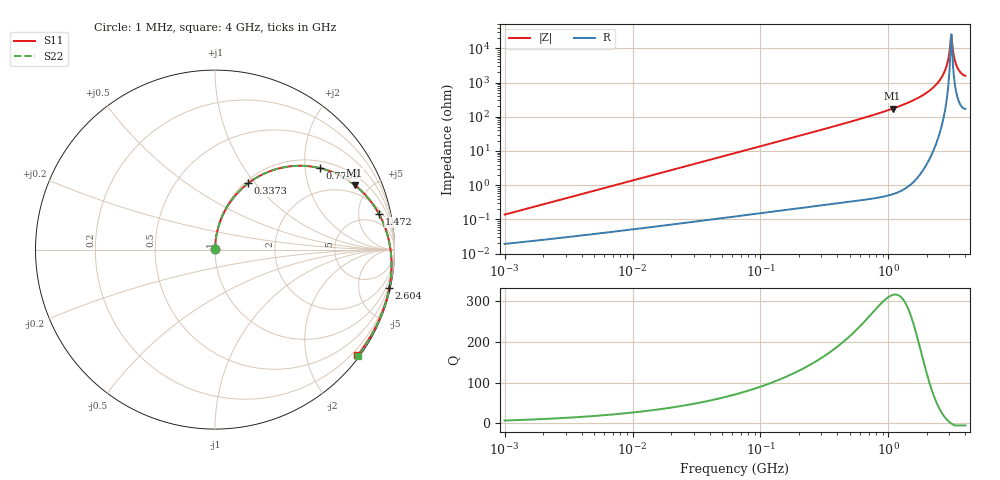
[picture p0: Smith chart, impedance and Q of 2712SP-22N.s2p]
# MHz  S  MA  R  50
!Freq  MagS11  AngS11  MagS21  AngS21  MagS12  AngS12  MagS22  AngS22
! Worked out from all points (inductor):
!   801 points, 1 MHz to 4 GHz, reference 50 ohm
!   read as one part in series: L = 21.9 nH near 1.042 MHz
!   highest Q = 316 at 1.078 GHz (marker M1), where L = 25.4 nH
!   self-resonance near 3.075 GHz
!   S11 on the Smith chart (normalised r, x): 1 MHz: 1.00, +0.00; 337.3 MHz: 1.04, +0.92; 773.6 MHz: 1.20, +2.41; 1.472 GHz: 2.68, +8.46; 2.604 GHz: 0.24, -9.18; 4 GHz: 0.06, -3.02
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1  0.00134 81.6  0.9998 -0.1  0.9998 -0.1  0.00134 81.6
4.016383  0.005336 86.0  0.9996 -0.3  0.9996 -0.3  0.005336 86.0
15.96482  0.02117 87.0  0.9991 -1.3  0.9991 -1.3  0.02116 87.0
63.45894  0.08382 84.0  0.9953 -5.1  0.9953 -5.1  0.08381 84.0
252.2445  0.3189 69.6  0.9455 -20.0  0.9455 -20.0  0.3188 69.6
337.2844  0.4124 63.5  0.9085 -26.2  0.9085 -26.2  0.4123 63.5
543.6043  0.5982 50.1  0.7987 -39.7  0.7987 -39.7  0.598 50.1
773.5614  0.7415 37.7  0.6683 -52.1  0.6683 -52.1  0.7412 37.7
1013.11  0.8378 27.3  0.5436 -62.5  0.5436 -62.5  0.8373 27.3
1078.187  0.8571 24.9  0.5126 -64.9  0.5126 -64.9  0.8567 24.9
1471.91  0.9349 12.3  0.3519 -77.5  0.3519 -77.5  0.9344 12.3
2094.561  0.9834 -2.6  0.1716 -92.0  0.1716 -92.0  0.9832 -2.6
2604.497  0.9945 -12.4  0.0699 -100.3  0.0699 -100.3  0.9948 -12.4
2829.918  0.9955 -16.4  0.03506 -101.3  0.03506 -101.3  0.9962 -16.4
2919.392  0.9956 -18.0  0.02285 -99.6  0.02285 -99.6  0.9964 -18.0
3011.696  0.9954 -19.6  0.01136 -91.4  0.01136 -91.4  0.9964 -19.6
3106.919  0.9951 -21.2  0.003799 -14.4  0.003799 -14.4  0.9962 -21.2
3205.151  0.9946 -22.9  0.01175 47.1  0.01175 47.1  0.996 -22.9
3340.977  0.9938 -25.2  0.02439 54.5  0.02439 54.5  0.9954 -25.2
3482.558  0.9928 -27.6  0.03569 54.8  0.03569 54.8  0.9948 -27.6
3706.259  0.9911 -31.4  0.04897 52.4  0.04897 52.4  0.9937 -31.4
4000  0.989 -36.6  0.05688 47.3  0.05688 47.3  0.9927 -36.6
